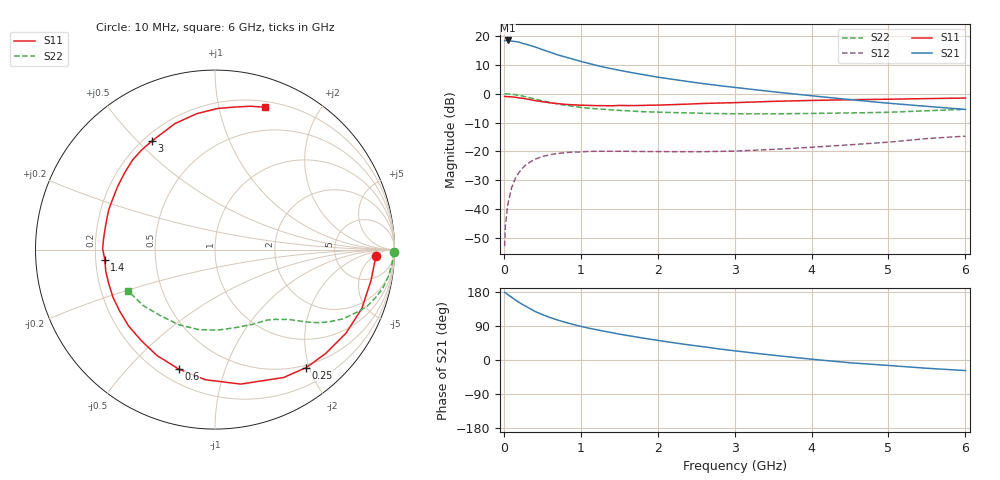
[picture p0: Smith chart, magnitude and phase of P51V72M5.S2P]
! SIEMENS Small Signal Semiconductors
! BFP183
! Si NPN RF Bipolar Junction Transistor in SOT143
! VCE = 1.75 V  IC = 2.5 mA
! Common Emitter S-Parameters:  March  1996
# GHz  S  MA  R  50
!  f  S11  S21  S12  S22
! GHz  MAG  ANG  MAG  ANG  MAG  ANG  MAG  ANG
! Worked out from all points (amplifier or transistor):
!   36 points, 10 MHz to 6 GHz, reference 50 ohm
!   highest |S21| = 18.4 dB at 50 MHz (marker M1)
!   |S21| within 3 dB of that: start of sweep to 483.3 MHz
!   unconditionally stable (mu >= 1): 1.935 GHz to 5.928 GHz
!   at 250 MHz: K = 0.14, MSG = 21.5 dB, |S12| = -25.5 dB
!   at 1.4 GHz: K = 0.74, MSG = 14.3 dB, |S12| = -19.9 dB
!   at 6 GHz: K = 0.99, MSG = 4.6 dB, |S12| = -14.7 dB
!   S11 on the Smith chart (normalised r, x): 10 MHz: 17, -6; 250 MHz: 0.46, -1.95; 600 MHz: 0.27, -0.70; 1.4 GHz: 0.24, -0.04; 3 GHz: 0.23, +0.55; 6 GHz: 0.25, +1.38
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0.01  0.8999 -2.3  8.268 178.8  0.0023 88.1  0.9973 -0.8
0.02  0.892 -4.7  8.296 177.6  0.0051 85.6  0.9941 -1.8
0.05  0.8861 -11.2  8.338 172.8  0.0118 86.0  0.9898 -4.4
0.1  0.8815 -21.9  8.112 165.7  0.0233 77.7  0.978 -8.7
0.2  0.8456 -43.3  7.784 151.7  0.044 66.6  0.9335 -16.7
0.25  0.8307 -52.3  7.379 145.6  0.0528 61.3  0.9052 -20.3
0.3  0.8087 -61.8  7.105 140.1  0.0608 56.9  0.8733 -23.1
0.4  0.7628 -79.2  6.476 128.8  0.0729 48.4  0.811 -28.4
0.5  0.727 -94.3  5.794 119.8  0.0818 41.7  0.7529 -32.3
0.6  0.6955 -106.9  5.233 112.2  0.0881 36.5  0.7064 -35.2
0.7  0.6729 -118.7  4.694 105.5  0.0922 32.0  0.665 -37.5
0.8  0.6527 -129.0  4.312 99.3  0.0956 28.6  0.6327 -39.3
0.9  0.6426 -138.4  3.954 93.9  0.0978 25.7  0.6029 -41.0
1.1  0.6274 -155.0  3.352 84.1  0.1002 21.1  0.5611 -43.9
1.4  0.6165 -174.7  2.704 72.3  0.1011 16.4  0.5253 -47.9
1.8  0.6266 164.1  2.152 58.1  0.1 14.6  0.4891 -53.4
2.2  0.6467 147.0  1.766 45.7  0.0993 14.0  0.4714 -60.0
3  0.6997 120.1  1.285 24.2  0.1016 17.7  0.4489 -76.1
3.5  0.7368 107.6  1.08 12.6  0.1086 20.7  0.4486 -87.6
4.5  0.7865 88.9  0.79 -7.3  0.1306 23.2  0.4643 -115.5
5.5  0.8224 76.2  0.604 -21.8  0.1672 21.8  0.507 -142.0
6  0.8405 70.8  0.534 -27.9  0.1843 18.3  0.536 -154.5
